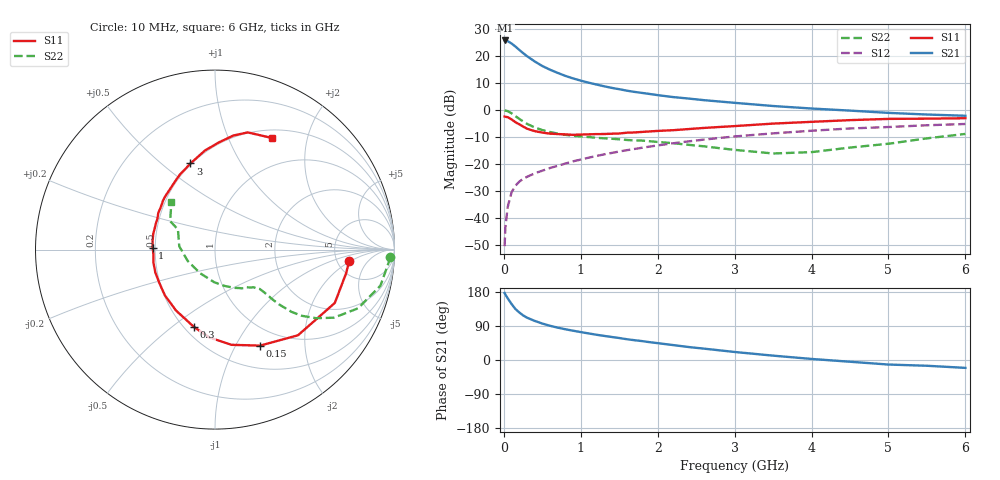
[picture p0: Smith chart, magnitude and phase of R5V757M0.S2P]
! SIEMENS Small Signal Semiconductors
! BFR183
! Si NPN RF Bipolar Junction Transistor in SOT23
! VCE = 0.75 V  IC = 7 mA
! Common Emitter S-Parameters:  May  1996
# GHz  S  MA  R  50
!  f  S11  S21  S12  S22
! GHz  MAG  ANG  MAG  ANG  MAG  ANG  MAG  ANG
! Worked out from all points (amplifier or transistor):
!   36 points, 10 MHz to 6 GHz, reference 50 ohm
!   highest |S21| = 25.6 dB at 20 MHz (marker M1)
!   |S21| within 3 dB of that: start of sweep to 181 MHz
!   unconditionally stable (mu >= 1): 804.9 MHz to 2.964 GHz
!   at 250 MHz: K = 0.53, MSG = 23.3 dB, |S12| = -25.6 dB
!   at 1.4 GHz: K = 1.08, MAG = 10.3 dB, |S12| = -16.0 dB
!   at 6 GHz: K = 0.95, MSG = 1.5 dB, |S12| = -5.3 dB
!   S11 on the Smith chart (normalised r, x): 10 MHz: 6.43, -1.88; 150 MHz: 0.77, -1.26; 300 MHz: 0.56, -0.60; 1 GHz: 0.48, +0.01; 3 GHz: 0.49, +0.63; 6 GHz: 0.60, +1.45
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0.01  0.7496 -4.9  19 176.7  0.003 85.8  0.9785 -2.4
0.02  0.7428 -10.0  19.15 172.8  0.0067 85.1  0.9671 -5.0
0.05  0.7308 -24.0  18.58 162.8  0.0159 78.1  0.9434 -12.3
0.1  0.6646 -45.9  16.83 147.9  0.0296 69.8  0.8618 -22.3
0.15  0.5912 -64.8  14.8 134.7  0.0393 62.5  0.7634 -29.8
0.2  0.5386 -80.1  12.85 125.6  0.0467 58.8  0.6798 -34.2
0.25  0.4907 -93.7  11.19 117.8  0.0527 56.4  0.6085 -37.3
0.3  0.4467 -105.2  9.839 111.8  0.0574 55.3  0.551 -39.1
0.4  0.403 -122.6  7.857 103.3  0.0666 54.9  0.4715 -40.5
0.5  0.3786 -137.3  6.447 96.2  0.0747 55.2  0.4218 -40.9
0.6  0.3616 -149.2  5.513 90.3  0.0836 56.1  0.3876 -40.9
0.8  0.3504 -168.0  4.235 81.1  0.1012 57.3  0.3443 -41.2
1  0.3479 178.1  3.459 73.6  0.1199 57.7  0.3217 -42.0
1.1  0.3509 171.9  3.178 70.2  0.1298 57.8  0.3131 -43.2
1.3  0.3559 161.2  2.726 63.7  0.1493 57.3  0.2967 -45.0
1.6  0.3768 146.9  2.255 54.8  0.179 55.9  0.2763 -49.6
2.2  0.4191 126.9  1.718 39.4  0.24 51.1  0.241 -62.3
3  0.4991 105.9  1.344 21.2  0.321 42.0  0.1814 -91.6
3.5  0.555 95.8  1.174 11.5  0.3662 35.4  0.1554 -122.1
4.5  0.6434 80.9  0.965 -4.6  0.4513 22.5  0.2 174.7
5.5  0.685 68.4  0.817 -15.2  0.517 10.7  0.2961 147.6
6  0.6976 63.1  0.775 -20.8  0.5459 3.1  0.3577 132.8
